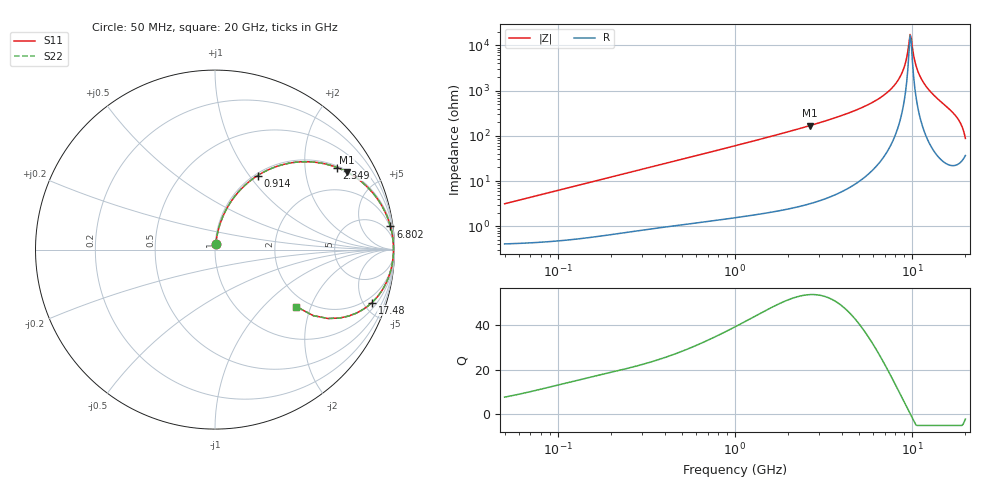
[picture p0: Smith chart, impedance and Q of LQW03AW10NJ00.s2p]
!Murata Part Number: LQW03AW10NJ00
!These Parameters are Measured in Series Mode Connection
!  o--[Z]--o
!Port1  Port2
!  o-------o
!Freq. Start=50[MHz] Stop=20[GHz], 401[Steps]
# Hz S RI R 50
!Freq.(Hz) S11(Real) S11(Imag) S21(Real) S21(Imag) S12(Real) S12(Imag) S22(Real) S22(Imag)
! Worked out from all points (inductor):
!   401 points, 50 MHz to 20 GHz, reference 50 ohm
!   read as one part in series: L = 9.88 nH near 51.52 MHz
!   highest Q = 53.6 at 2.647 GHz (marker M1), where L = 10.1 nH
!   self-resonance near 9.745 GHz
!   S11 on the Smith chart (normalised r, x): 50 MHz: 1.01, +0.06; 914 MHz: 1.03, +1.10; 2.349 GHz: 1.06, +2.94; 6.802 GHz: 2, +15; 17.48 GHz: 1.44, -5.75; 20 GHz: 1.73, -1.59
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5e7  0.00499 0.0308  0.995 -0.0308  0.995 -0.0308  0.00499 0.0308
1.364002e8  0.0122 0.0827  0.9878 -0.0827  0.9878 -0.0827  0.0122 0.0827
3.721004e8  0.0562 0.2109  0.9438 -0.2109  0.9438 -0.2109  0.0562 0.2109
9.140482e8  0.2381 0.4128  0.7619 -0.4128  0.7619 -0.4128  0.2381 0.4128
1e9  0.2711 0.432  0.7289 -0.432  0.7289 -0.432  0.2711 0.432
2.348516e9  0.6805 0.457  0.3195 -0.457  0.3195 -0.457  0.6805 0.457
2.647493e9  0.7352 0.432  0.2648 -0.432  0.2648 -0.432  0.7352 0.432
2.728004e9  0.7481 0.4249  0.2519 -0.4249  0.2519 -0.4249  0.7481 0.4249
4.677679e9  0.9207 0.2589  0.0793 -0.2589  0.0793 -0.2589  0.9207 0.2589
6.802353e9  0.9775 0.129  0.0225 -0.129  0.0225 -0.129  0.9775 0.129
7.442007e9  0.985 0.0976  0.015 -0.0976  0.015 -0.0976  0.985 0.0976
8.774992e9  0.9931 0.0395  0.00691 -0.0395  0.00691 -0.0395  0.9931 0.0395
9.178299e9  0.9941 0.0233  0.00593 -0.0233  0.00593 -0.0233  0.9941 0.0233
9.600142e9  0.9945 0.00703  0.00549 -0.00703  0.00549 -0.00703  0.9945 0.00703
9.745021e9  0.9945 0.00155  0.00547 -0.00155  0.00547 -0.00155  0.9945 0.00155
1.004137e10  0.9944 -0.0095  0.00562 0.0095  0.00562 0.0095  0.9944 -0.0095
1.066139e10  0.9933 -0.032  0.00673 0.032  0.00673 0.032  0.9933 -0.032
1.166392e10  0.9893 -0.0672  0.0107 0.0672  0.0107 0.0672  0.9893 -0.0672
1.314879e10  0.9785 -0.1182  0.0215 0.1182  0.0215 0.1182  0.9785 -0.1182
1.747767e10  0.8747 -0.2948  0.1253 0.2948  0.1253 0.2948  0.8747 -0.2948
1.855685e10  0.7835 -0.3557  0.2165 0.3557  0.2165 0.3557  0.7835 -0.3557
2e10  0.4531 -0.318  0.5469 0.318  0.5469 0.318  0.4531 -0.318
